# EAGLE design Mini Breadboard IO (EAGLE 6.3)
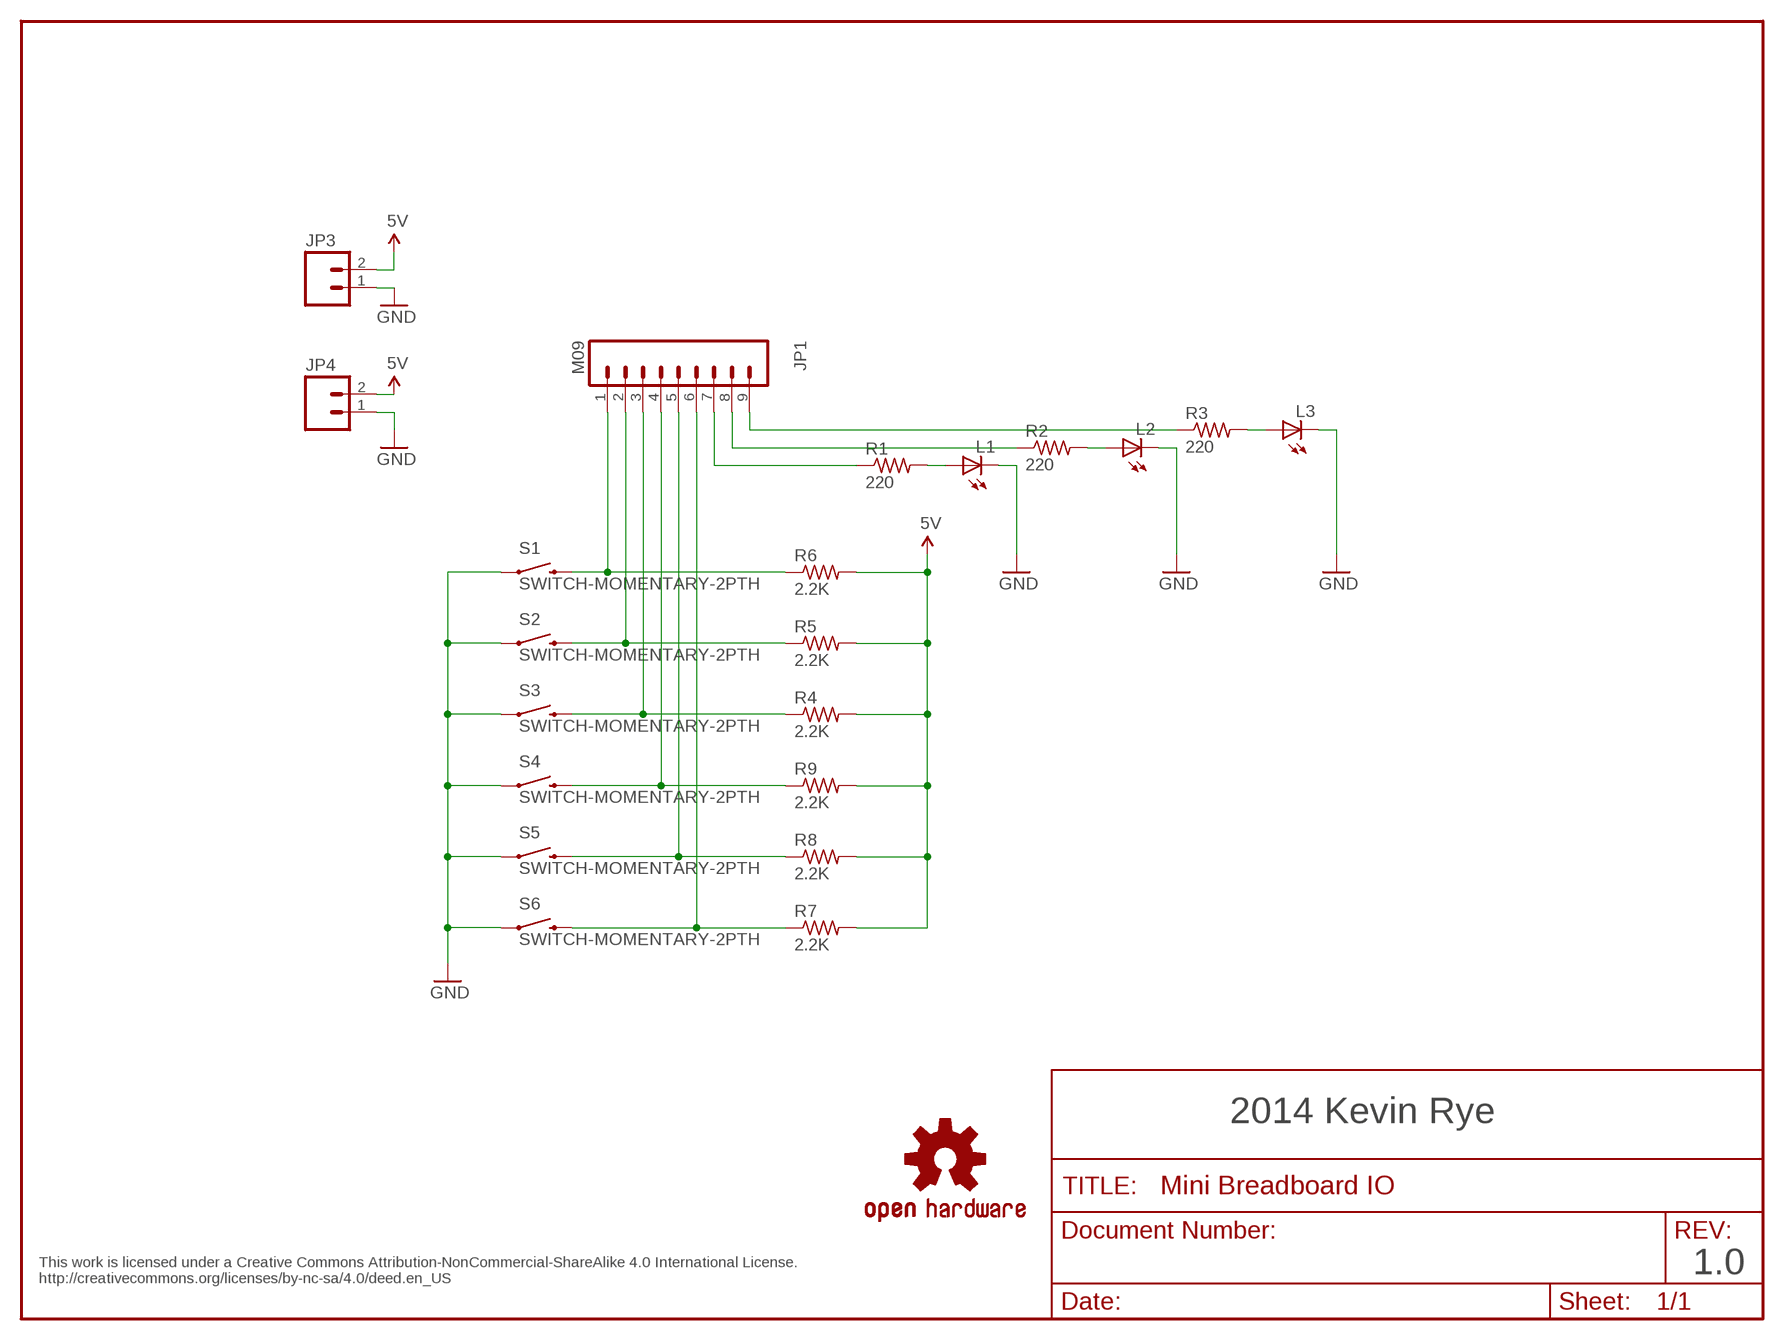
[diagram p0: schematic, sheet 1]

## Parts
JP1  M09  [1X09]
JP3  M02PTH  [1X02]
JP4  M02PTH  [1X02]
L1  LED0603  [LED-0603]
L2  LED0603  [LED-0603]
L3  LED0603  [LED-0603]
R1  220  R-US_R0805  [R0805]
R2  220  R-US_R0805  [R0805]
R3  220  R-US_R0805  [R0805]
R4  2.2K  R-US_R0805  [R0805]
R5  2.2K  R-US_R0805  [R0805]
R6  2.2K  R-US_R0805  [R0805]
R7  2.2K  R-US_R0805  [R0805]
R8  2.2K  R-US_R0805  [R0805]
R9  2.2K  R-US_R0805  [R0805]
S1  SWITCH-MOMENTARY-2PTH  [TACTILE-PTH]
S2  SWITCH-MOMENTARY-2PTH  [TACTILE-PTH]
S3  SWITCH-MOMENTARY-2PTH  [TACTILE-PTH]
S4  SWITCH-MOMENTARY-2PTH  [TACTILE-PTH]
S5  SWITCH-MOMENTARY-2PTH  [TACTILE-PTH]
S6  SWITCH-MOMENTARY-2PTH  [TACTILE-PTH]
U$7  OSHW-LOGOS  [OSHW-LOGO-S]

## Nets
5V: JP3.2 JP4.2 R4.2 R5.2 R6.2 R7.2 R8.2 R9.2
GND: JP3.1 JP4.1 L1.C L2.C L3.C S1.1 S2.1 S3.1 S4.1 S5.1 S6.1
N$2: JP1.6 R7.1 S6.3
N$3: JP1.5 R8.1 S5.3
N$4: JP1.4 R9.1 S4.3
N$5: JP1.3 R4.1 S3.3
N$6: JP1.2 R5.1 S2.3
N$7: JP1.1 R6.1 S1.3
N$8: JP1.7 R1.1
N$9: JP1.8 R2.1
N$10: JP1.9 R3.1
N$13: L3.A R3.2
N$14: L2.A R2.2
N$15: L1.A R1.2

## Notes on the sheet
- 2014 Kevin Rye
- 1.0
- This work is licensed under a Creative Commons Attribution-NonCommercial-ShareAlike 4.0 International License.
  http://creativecommons.org/licenses/by-nc-sa/4.0/deed.en_US

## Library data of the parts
JP1 = SparkFun w:epaper:M09: Header 9 Standard 9-pin 0.1" header. Use with straight break away headers (SKU : PRT-00116), right angle break away headers (PRT-00553), swiss pins (PRT-00743), machine pins (PRT-00117), and female headers (PRT-00115).
JP3 JP4 = SparkFun-Connectors:M02: Header 2
L1-L3 = SparkFun-LED:LED: LEDs
R1-R9 = adafruit:R-US_: RESISTOR, American symbol
S1-S6 = SparkFun:SWITCH-MOMENTARY-2
U$7 = SparkFun:OSHW-LOGO: Open Source Hardware Logo This logo indicates the piece of hardware it is found on incorporates a OSHW license and/or adheres to the definition of open source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

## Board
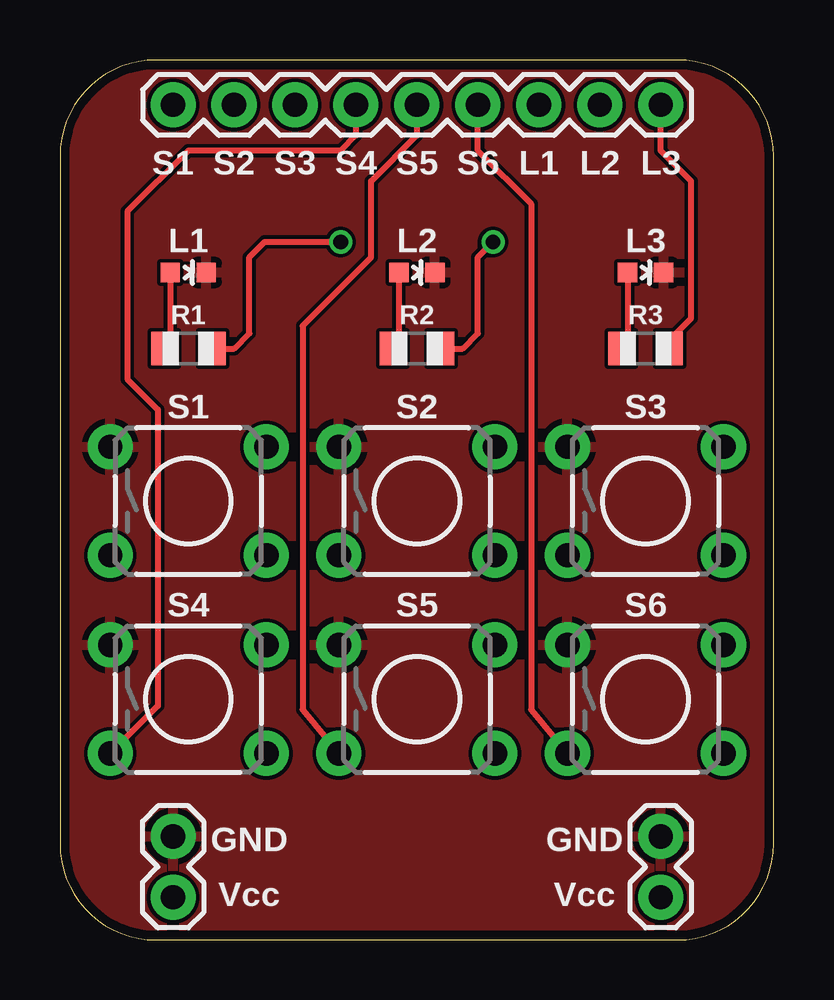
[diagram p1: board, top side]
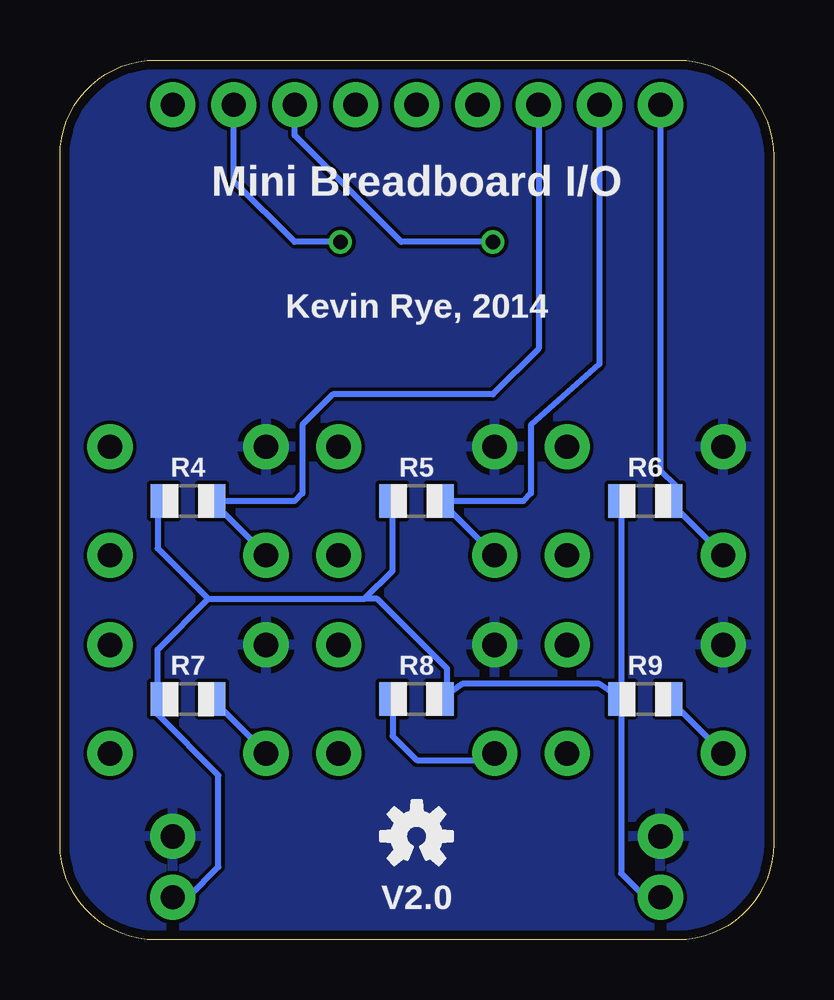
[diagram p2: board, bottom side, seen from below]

Size 29.73 x 36.66 mm. Coordinates in mm from the lower left corner, seen from the top.
Copper layers (1*16): Top 0.0356mm / dielectric 1.5011mm / Bottom 0.0356mm
Design rules "LaenPCBOrder": minimum track width 6mil, minimum drill 13mil, track to track 6mil, track to pad 6mil, pad to pad 6mil, via to via 6mil, smd to smd 6mil, copper to edge 15mil, drill to drill 6mil, minimum pad ring 7mil, minimum via ring 7mil, stop-mask expansion 3mil, vias tented up to drill 0mil, thermal gap 10mil

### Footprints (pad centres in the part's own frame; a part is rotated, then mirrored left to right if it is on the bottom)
1X09 = drill 1.016 pad 1.88: 1 0,0; 2 2.54,0; 3 5.08,0; 4 7.62,0; 5 10.16,0; 6 12.7,0; 7 15.24,0; 8 17.78,0; 9 20.32,0
1X02 = drill 1.016 pad 1.88: 1 0,0; 2 2.54,0
LED-0603 = smd 0.8 x 0.8: A 0,-0.75; C 0,0.75
R0805 = smd 1.1 x 1.4: 1 -1,0; 2 1,0
TACTILE-PTH = drill 1.016 pad 1.88: 1 -3.251,2.261; 2 3.251,2.261; 3 -3.251,-2.261; 4 3.251,-2.261

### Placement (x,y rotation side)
JP1  4.71,34.8 0 top
JP3  4.71,4.32 270 top
JP4  25.03,4.32 270 top
L1  5.35,27.81 270 top
L2  14.87,27.81 270 top
L3  24.4,27.81 270 top
R1  5.35,24.64 180 top
R2  14.87,24.64 180 top
R3  24.4,24.64 180 top
R4  24.4,18.29 180 bottom
R5  14.87,18.29 180 bottom
R6  5.35,18.29 180 bottom
R7  24.4,10.03 180 bottom
R8  14.87,10.03 0 bottom
R9  5.35,10.03 180 bottom
S1  5.35,18.29 0 top
S2  14.87,18.29 0 top
S3  24.4,18.29 0 top
S4  5.35,10.03 0 top
S5  14.87,10.03 0 top
S6  24.4,10.03 0 top
U$2  [DP50XX_BUTTONBREAKOUT2]  0.52,0 0 top
U$7  14.87,4.32 0 bottom

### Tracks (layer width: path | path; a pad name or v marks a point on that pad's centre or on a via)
5V
  Bottom 0.254: 16.14,18.02 R5.2 15.87,15.38 17.05,14.21 | R9.2 6.62,9.76 | R4.2 25.67,18.02 25.67,16.32 23.56,14.21 | 23.56,14.21 17.05,14.21 | R6.2 R9.2 | JP3.2 5.35,1.78 6.35,2.78 R9.2 | JP4.2 24.4,1.78 23.13,3.05 23.13,6.86 25.67,9.4 25.67,9.76 R7.2 25.67,10.3 25.67,12.1 23.56,14.21 | R9.2 7.25,10.67 12.97,10.67 R8.2 13.6,10.03 13.6,11.3 16.51,14.21 17.05,14.21
GND
  pour Top: -2.27,38.61 32.02,38.61 32.02,-2.03 -2.27,-2.03
  pour Bottom: -1.64,37.34 30.11,37.34 30.75,-0.76 -1,-0.76
N$2
  Top 0.254: S6.3 19.63,9.6 19.63,30.67 17.41,32.89 JP1.6
  Bottom 0.254: S6.3 21.15,7.78 R7.1
N$3
  Top 0.254: JP1.5 14.87,33.53 12.97,31.62 12.97,28.45 10.11,25.59 10.11,9.6 S5.3
  Bottom 0.254: R8.1 15.87,8.49 14.87,7.49 11.9,7.49 S5.3
N$4
  Top 0.254: JP1.4 12.33,33.53 11.7,32.89 5.35,32.89 2.81,30.35 2.81,23.37 4.08,22.1 4.08,9.75 S4.3
  Bottom 0.254: R9.1 S4.3
N$5
  Bottom 0.254: JP1.3 9.79,24.64 11.7,22.73 18.36,22.73 19.63,21.46 19.63,18.61 19.95,18.29 R4.1 S3.3
N$6
  Bottom 0.254: JP1.2 7.25,24 10.11,21.46 10.11,18.61 10.43,18.29 R5.1 S2.3
N$7
  Bottom 0.254: JP1.1 4.71,19.56 4.08,18.92 4.08,18.56 R6.1 S1.3 2.17,16.1
N$8  (via drill 0.61)
  Top 0.254: R1.1 7.25,24.64 7.89,25.27 7.89,28.45 8.52,29.08 v11.7,29.08
  Bottom 0.254: v11.7,29.08 15.51,29.08 19.95,33.53 JP1.7
N$9  (via drill 0.61)
  Top 0.254: R2.1 16.78,24.64 17.41,25.27 17.41,28.45 v18.05,29.08
  Bottom 0.254: v18.05,29.08 19.95,29.08 22.49,31.62 JP1.8
N$10
  Top 0.254: R3.1 25.4,25 26.3,25.91 26.3,31.62 25.03,32.89 JP1.9
N$13
  Top 0.254: L3.A 23.65,24.89 R3.2
N$14
  Top 0.254: L2.A 14.12,24.89 R2.2
N$15
  Top 0.254: L1.A 4.6,24.89 R1.2

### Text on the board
Unrouted: This work is licensed under a Creative Commons Attribution-NonCommercial-ShareAlike 4.0 International License. / http://creativecommons.org/licenses/by-nc-sa/4.0/deed.en_US
tNames: S1 | S2 | S3 | S4 | S5 | S6 | L1 | L2 | L3 | GND | GND | Vcc | Vcc
bNames: Mini Breadboard I/O | Kevin Rye, 2014 | V2.0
